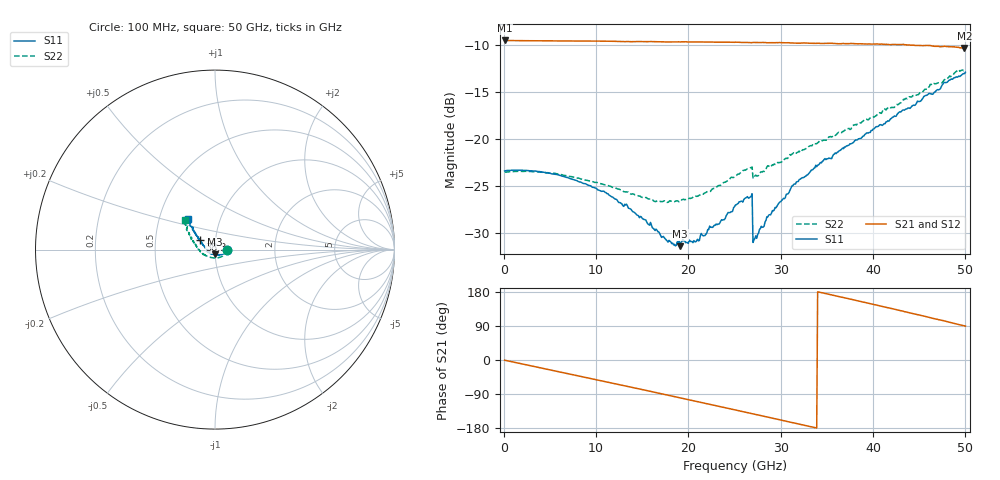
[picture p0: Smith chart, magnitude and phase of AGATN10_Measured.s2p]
! Filename4Jim: AG16_W2_AGATN10_A_1015_LRM_1BW_LRM.s2p
! Calibration: AG02 LRM + TRL
! Notes:
! Row:10, Col:15
! Probes: nan
! Prober: MPI TS150
! Date: 2023-09-21 15:16:17
! DC: None
# GHz S dB R 50
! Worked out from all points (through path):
!   500 points, 100 MHz to 50 GHz, reference 50 ohm
!   highest |S21| = -9.51 dB at 100 MHz (marker M1); lowest = -10.3 dB at 49.9 GHz (marker M2)
!   group delay of S21, straight-line fit = 15 ps
!   lowest |S11| = -31.4 dB at 19.1 GHz (marker M3), VSWR 1.06, Z = 49.7 - j2.66 ohm
!   |S11| at or under -10 dB: start of sweep to end of sweep
!   |S22| runs from -26.8 to -12.6 dB; largest |S21 - S12| = 0.0013
!   S11 on the Smith chart (normalised r, x): 100 MHz: 1.15, +0.00; 38.3 GHz: 0.84, +0.09; 50 GHz: 0.70, +0.25
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0.1  -23.40 0.0  -9.51 -0.6  -9.50 -0.6  -23.55 0.0
4.3  -23.54 -7.6  -9.55 -22.3  -9.54 -22.3  -23.54 -11.2
8.5  -24.68 -18.5  -9.58 -44.1  -9.57 -44.1  -24.29 -26.1
13.3  -26.95 -38.4  -9.63 -69.1  -9.62 -69.2  -25.64 -51.9
16.8  -29.88 -69.0  -9.65 -87.6  -9.64 -87.6  -26.60 -80.2
18.4  -31.27 -87.2  -9.66 -95.9  -9.66 -96.0  -26.65 -95.2
19.1  -31.42 -95.0  -9.67 -99.6  -9.66 -99.7  -26.69 -101.4
21  -30.67 -124.0  -9.67 -109.8  -9.66 -109.9  -26.10 -120.5
22.3  -29.29 -139.6  -9.68 -116.7  -9.67 -116.8  -25.60 -131.5
23.9  -28.60 -155.5  -9.68 -125.4  -9.67 -125.5  -24.60 -143.6
25.1  -27.03 -163.9  -9.69 -131.9  -9.68 -131.9  -23.96 -151.9
26.7  -26.19 -174.7  -9.73 -140.6  -9.73 -140.6  -23.06 -161.5
27.2  -30.60 -166.8  -9.72 -143.2  -9.71 -143.3  -23.95 -150.1
28.6  -28.29 -178.1  -9.75 -150.7  -9.75 -150.8  -22.85 -159.1
31.3  -25.00 168.8  -9.78 -165.5  -9.77 -165.6  -21.56 -173.0
33.4  -23.30 159.4  -9.81 -176.8  -9.80 -176.9  -20.71 178.0
38.3  -20.10 148.0  -9.87 156.3  -9.86 156.1  -18.39 162.9
41.7  -18.11 143.1  -9.94 137.4  -9.93 137.2  -16.64 154.1
46.1  -15.14 135.4  -10.05 112.2  -10.04 112.0  -14.41 145.7
49.1  -13.43 130.0  -10.24 94.5  -10.23 94.4  -12.75 137.4
49.9  -13.05 130.3  -10.32 90.1  -10.32 89.9  -12.65 135.4
50  -12.89 130.8  -10.32 89.6  -10.31 89.4  -12.64 135.4
